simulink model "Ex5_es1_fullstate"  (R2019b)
settings: Solver=FixedStepDiscrete  StartTime=0  StopTime=20  FixedStep=1  RelTol=1e-3
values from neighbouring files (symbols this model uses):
  A = [ 0.5 1; 0 0.5 ]    [ScriptCD_Es01.m]
  B = [0;0]    [ScriptCD_Es01.m]
  C = [1 0]    [ScriptCD_Es01.m]
  x10 = 2    [ScriptCD_Es01.m]
  x20 = -11    [ScriptCD_Es01.m]

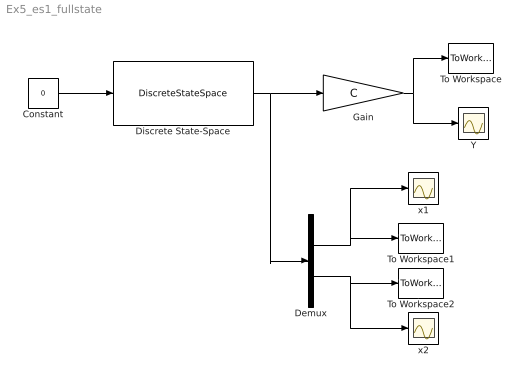
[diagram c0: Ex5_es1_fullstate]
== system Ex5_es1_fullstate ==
  Constant : Constant  Value=0
  Demux : Demux  Outputs=2
  Discrete State-Space : DiscreteStateSpace  A=A  B=B  C=eye(2)  D=zeros(2,1)  InitialCondition=[x10;x20]
  Gain : Gain  Gain=C  Multiplication=Matrix(K*u)
  To Workspace : ToWorkspace  VariableName=y  SaveFormat=Timeseries  SampleTime=-1
  To Workspace1 : ToWorkspace  VariableName=x1  SaveFormat=Timeseries  SampleTime=-1
  To Workspace2 : ToWorkspace  VariableName=x2  SaveFormat=Timeseries  SampleTime=-1
  Y : Scope
  x1 : Scope
  x2 : Scope
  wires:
  Discrete State-Space/1 -> Demux/1, Gain/1
  Constant/1 -> Discrete State-Space/1
  Gain/1 -> To Workspace/1, Y/1
  Demux/1 -> x1/1, To Workspace1/1
  Demux/2 -> To Workspace2/1, x2/1
